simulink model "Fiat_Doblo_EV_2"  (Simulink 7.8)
settings: Solver=ode23t  StartTime=0.0  StopTime=1180  MaxStep=0.01  RelTol=1e-3
InitFcn:
  | init_FIAT_Doblo_EV
StopFcn:
  | Vyhodnoceni
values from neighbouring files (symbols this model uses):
  om_diff_ic = 0    [init_FIAT_Doblo_EV.m]
  omric = 0    [init_FIAT_Doblo_EV.m]
  t_sample = 0.1    [init_FIAT_Doblo_EV.m]
  vf0 = 0    [init_FIAT_Doblo_EV.m]
undefined symbols (not defined in the file or in its folder): Battery, Battery_Pack, BatteryData, Differential, Driveshaft, Environment, Gearbox, Motor, Powertrain, Vehicle
libraries: simulink x7, simulink_need_slupdate x1, simulink_extras x1

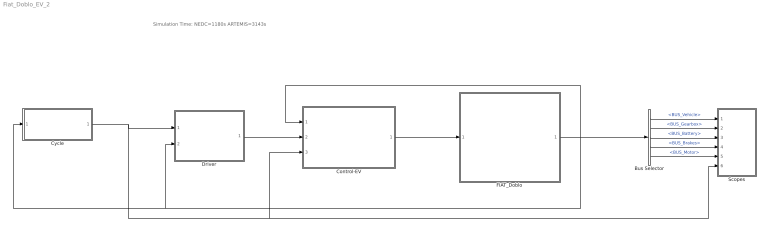
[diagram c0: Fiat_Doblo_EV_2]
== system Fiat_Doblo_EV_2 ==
  note: Simulation Time: NEDC=1180s ARTEMIS=3143s
  Bus Selector : BusSelector  OutputSignals=BUS_Vehicle,BUS_Gearbox,BUS_Battery,BUS_Brakes,BUS_Motor
  Control-EV : Subsystem
  Cycle : Subsystem
  Driver : Subsystem
  FIAT_Doblo : Subsystem
  Scopes : Subsystem
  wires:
  Control-EV/1(BUS_Control) -> FIAT_Doblo/1(BUS_Control)
  FIAT_Doblo/1(BUS_FIAT_Doblo) -> Bus Selector/1, Control-EV/1(BUS_FIAT_Doblo), Driver/2(BUS_FIAT_Doblo), Cycle/1(BUS_FIAT Doblo)
  Bus Selector/1 -> Scopes/1(BUS_Vehicle)  "<BUS_Vehicle>"
  Bus Selector/2 -> Scopes/2(BUS_Gearbox)  "<BUS_Gearbox>"
  Bus Selector/3 -> Scopes/3(BUS_Battery)  "<BUS_Battery>"
  Bus Selector/4 -> Scopes/4(BUS_Brakes)  "<BUS_Brakes>"
  Bus Selector/5 -> Scopes/5(BUS_Motor)  "<BUS_Motor>"
  Cycle/1(BUS_Cycle) -> Driver/1(BUS_Cycle), Scopes/6(BUS_Cycle), Control-EV/3(BUS_Cycle)
  Driver/1(BUS_Driver) -> Control-EV/2(BUS_Driver)

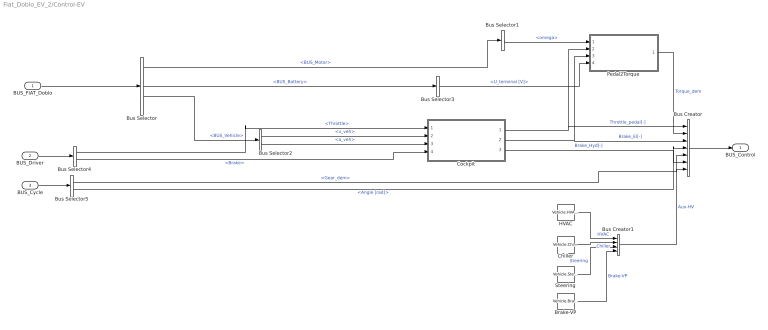
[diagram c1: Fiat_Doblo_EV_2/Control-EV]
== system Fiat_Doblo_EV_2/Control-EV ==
  BUS_FIAT_Doblo : Inport
  BUS_Driver : Inport  Port=2
  BUS_Cycle : Inport  Port=3
  Brake-VP : Constant  Value=Vehicle.BrakeVP.On
  Bus Creator : BusCreator  Inputs=7
  Bus Creator1 : BusCreator
  Bus Selector : BusSelector  OutputSignals=BUS_Motor,BUS_Gearbox,BUS_Battery,BUS_Vehicle,BUS_Brakes
  Bus Selector1 : BusSelector  OutputSignals=omega
  Bus Selector2 : BusSelector  OutputSignals=v_veh,a_veh
  Bus Selector3 : BusSelector  OutputSignals=U_terminal [V]
  Bus Selector4 : BusSelector  OutputSignals=Throttle,Brake
  Bus Selector5 : BusSelector  OutputSignals=Gear_dem,Angle [rad]
  Chiller : Constant  Value=Vehicle.Chiller.On
  Cockpit : Subsystem
  HVAC : Constant  Value=Vehicle.HVAC.On
  Pedal2Torque : Subsystem
  Steering : Constant  Value=Vehicle.Steering.On
  BUS_Control : Outport
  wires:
  Cockpit/1(Throttle1) -> Bus Creator/1, Pedal2Torque/2(Throttle_pedal[-])  "Throttle_pedal[-]"
  Cockpit/2(BrakeEl) -> Bus Creator/3, Pedal2Torque/3(Brake_el[-])  "Brake_El[-]"
  Bus Creator/1 -> BUS_Control/1
  Bus Selector2/1 -> Cockpit/2(v-veh)  "<v_veh>"
  Bus Selector2/2 -> Cockpit/3(a-veh)  "<a_veh>"
  Cockpit/3(BrakeHyd) -> Bus Creator/6  "Brake_Hyd[-]"
  HVAC/1 -> Bus Creator1/1  "HVAC"
  Chiller/1 -> Bus Creator1/2  "Chiller"
  Steering/1 -> Bus Creator1/3  "Steering"
  Brake-VP/1 -> Bus Creator1/4  "Brake-VP"
  Bus Creator1/1 -> Bus Creator/7  "Aux-HV"
  Bus Selector1/1 -> Pedal2Torque/1(om_motor)  "<omega>"
  Pedal2Torque/1(Te) -> Bus Creator/2  "Torque_dem"
  Bus Selector/3 -> Bus Selector3/1  "<BUS_Battery>"
  Bus Selector3/1 -> Pedal2Torque/4(Voltage [V])  "<U_terminal [V]>"
  BUS_FIAT_Doblo/1 -> Bus Selector/1
  Bus Selector/4 -> Bus Selector2/1  "<BUS_Vehicle>"
  Bus Selector/1 -> Bus Selector1/1  "<BUS_Motor>"
  BUS_Driver/1 -> Bus Selector4/1
  Bus Selector4/1 -> Cockpit/1(Throttle_in)  "<Throttle>"
  Bus Selector4/2 -> Cockpit/4(Brake)  "<Brake>"
  BUS_Cycle/1 -> Bus Selector5/1
  Bus Selector5/1 -> Bus Creator/5  "<Gear_dem>"
  Bus Selector5/2 -> Bus Creator/4  "<Angle [rad]>"

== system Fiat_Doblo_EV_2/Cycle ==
  BUS_FIAT Doblo : Inport
  Acc : Step  Time=15  After=250  SampleTime=0
  Bus Creator : BusCreator  Inputs=3
  Bus Selector : BusSelector  OutputSignals=BUS_Vehicle.s_veh
  Constant1 : Constant
  Constant2 : Constant  Value=2
  Constant4 : Constant  Value=0
  Demux1 : Demux  Outputs=2
  From File3 : FromFile  FileName=NEDC.mat  ExtrapolationBeforeFirstDataPoint=Hold first value  ExtrapolationAfterLastDataPoint=Hold last value  SampleTime=0.1
  From File4 : FromFile  FileName=artemis_mw130.mat  ExtrapolationBeforeFirstDataPoint=Hold first value  ExtrapolationAfterLastDataPoint=Hold last value  SampleTime=0.1
  From File5 : FromFile  FileName=artemis_URM150.mat  ExtrapolationBeforeFirstDataPoint=Hold first value  ExtrapolationAfterLastDataPoint=Hold last value  SampleTime=0.1
  Multiport Switch : MultiPortSwitch  Inputs=4  zeroidx=off
  Terminator1 : Terminator
  To Workspace : ToWorkspace  VariableName=v_dem  SampleTime=t_sample  SaveFormat=Array
  To Workspace2 : ToWorkspace  VariableName=Gear_dem  SampleTime=t_sample  SaveFormat=Array
  BUS_Cycle : Outport
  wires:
  Constant1/1 -> To Workspace2/1, Bus Creator/2  "Gear_dem"
  Bus Creator/1 -> BUS_Cycle/1
  Demux1/2 -> Terminator1/1
  Acc/1 -> Multiport Switch/5
  From File4/1 -> Multiport Switch/4
  From File5/1 -> Multiport Switch/3
  Demux1/1 -> Multiport Switch/2
  Multiport Switch/1 -> To Workspace/1, Bus Creator/1  "Speed_dem"
  Constant2/1 -> Multiport Switch/1
  From File3/1 -> Demux1/1
  BUS_FIAT Doblo/1 -> Bus Selector/1
  Constant4/1 -> Bus Creator/3  "Angle [rad]"

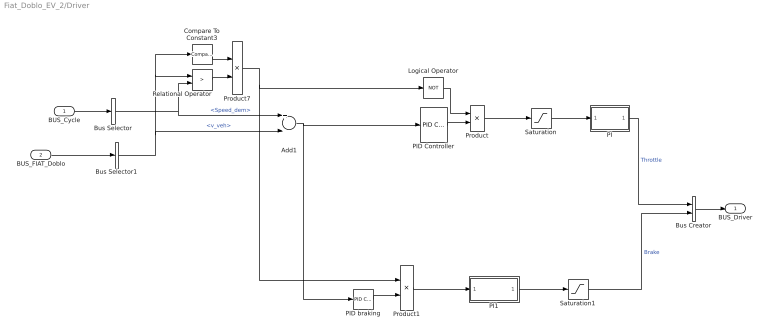
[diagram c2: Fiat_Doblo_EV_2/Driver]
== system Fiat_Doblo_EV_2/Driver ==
  BUS_Cycle : Inport
  BUS_FIAT_Doblo : Inport  Port=2
  Add1 : Sum  Inputs=+-
  Bus Creator : BusCreator  Inputs=2
  Bus Selector : BusSelector  OutputSignals=Speed_dem
  Bus Selector1 : BusSelector  OutputSignals=BUS_Vehicle.v_veh
  Compare To Constant3 : simulink/Logic and Bit Operations/Compare To Constant  relop=>  const=1  OutDataTypeStr=uint8  ZeroCross=off
  Logical Operator : Logic  Operator=NOT  AllPortsSameDT=off  OutDataTypeStr=boolean
  PI : Subsystem
  PI1 : Subsystem
  PID Controller : simulink/Continuous/PID Controller  Controller=PID  TimeDomain=Continuous-time  SampleTime=1  IntegratorMethod=Forward Euler  FilterMethod=Forward Euler  Form=Parallel  P=1  I=0.01  D=0  N=100  InitialConditionSource=internal  InitialConditionForIntegrator=0  InitialConditionForFilter=0  ExternalReset=none  LimitOutput=off  UpperSaturationLimit=1  LowerSaturationLimit=-1  LinearizeAsGain=off  AntiWindupMode=none  Kb=1  TrackingMode=off  Kt=1  PParamMin=[]  PParamMax=[]  IParamMin=[]  IParamMax=[]  DParamMin=[]  DParamMax=[]  NParamMin=[]  NParamMax=[]  KbParamMin=[]  KbParamMax=[]  KtParamMin=[]  KtParamMax=[]  POutMin=[]  POutMax=[]  IOutMin=[]  IOutMax=[]  DOutMin=[]  DOutMax=[]  NOutMin=[]  NOutMax=[]  KbOutMin=[]  KbOutMax=[]  KtOutMin=[]  KtOutMax=[]  IntegratorOutMin=[]  IntegratorOutMax=[]  FilterOutMin=[]  FilterOutMax=[]  SumOutMin=[]  SumOutMax=[]  SumI1OutMin=[]  SumI1OutMax=[]  SumI2OutMin=[]  SumI2OutMax=[]  SumI3OutMin=[]  SumI3OutMax=[]  SumDOutMin=[]  SumDOutMax=[]  SaturationOutMin=[]  SaturationOutMax=[]  IntegratorContinuousStateAttributes=''  IntegratorStateMustResolveToSignalObject=off  IntegratorRTWStateStorageClass=Auto  FilterContinuousStateAttributes=''  FilterStateMustResolveToSignalObject=off  FilterRTWStateStorageClass=Auto
  PID braking : simulink_need_slupdate/PID Controller  P=0.3  I=0.01  D=0
  Product : Product
  Product1 : Product
  Product7 : Product
  Relational Operator : RelationalOperator  Operator=>  OutDataTypeStr=boolean
  Saturation : Saturate  UpperLimit=1  LowerLimit=0
  Saturation1 : Saturate  UpperLimit=0  LowerLimit=-1
  BUS_Driver : Outport
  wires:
  PID braking/1 -> Product1/2
  Product1/1 -> PI1/1(In1)
  Add1/1 -> PID braking/1, PID Controller/1
  PID Controller/1 -> Product/2
  Product/1 -> Saturation/1
  Logical Operator/1 -> Product/1
  Saturation1/1 -> Bus Creator/2  "Brake"
  Product7/1 -> Product1/1, Logical Operator/1
  Compare To Constant3/1 -> Product7/1
  Relational Operator/1 -> Product7/2
  PI1/1(Out1) -> Saturation1/1
  Saturation/1 -> PI/1(In1)
  PI/1(Out1) -> Bus Creator/1  "Throttle"
  BUS_Cycle/1 -> Bus Selector/1
  Bus Selector/1 -> Relational Operator/2, Add1/1  "<Speed_dem>"
  BUS_FIAT_Doblo/1 -> Bus Selector1/1
  Bus Selector1/1 -> Compare To Constant3/1, Relational Operator/1, Add1/2  "<v_veh>"
  Bus Creator/1 -> BUS_Driver/1

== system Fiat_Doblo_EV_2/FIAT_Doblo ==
  BUS_Control : Inport
  01-Electric Motor : Subsystem  AncestorBlock=Powertrain/Electric Drive
  02-Gearbox : Subsystem  AncestorBlock=Powertrain/03-Gearbox
  03-Differential&Drive shaft : Subsystem  AncestorBlock=Powertrain/04-Differential&Drive shaft
  04-Vehicle : Subsystem  AncestorBlock=Powertrain/05-Vehicle
  05-Battery_Pack : Subsystem  AncestorBlock=Powertrain/Battery_Pack
  06-Hydraulic Brakes : Subsystem  AncestorBlock=Powertrain/Hydraulic Brakes  TreatAsAtomicUnit=on
  Bus Creator : BusCreator  Inputs=6
  Clock : Clock
  HV-Boardnet : Subsystem  TreatAsAtomicUnit=on
  To Workspace5 : ToWorkspace  VariableName=t  SampleTime=t_sample  SaveFormat=Array
  BUS_FIAT_Doblo : Outport
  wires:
  02-Gearbox/1(BUS_Gearbox) -> 03-Differential&Drive shaft/1(BUS_Gearbox), 01-Electric Motor/1(BUS_Gearbox), Bus Creator/2  "BUS_Gearbox"
  03-Differential&Drive shaft/1(BUS_Driveshaft) -> 02-Gearbox/2(BUS_Driveshaft), 04-Vehicle/1(BUS_Driveshaft_Front)
  04-Vehicle/1(BUS_Vehicle) -> 03-Differential&Drive shaft/2(BUS_Vehicle), Bus Creator/3  "BUS_Vehicle"
  05-Battery_Pack/1(BUS_Battery) -> 01-Electric Motor/3(BUS_Battery), Bus Creator/4  "BUS_Battery"
  06-Hydraulic Brakes/1(BUS_Brakes) -> 04-Vehicle/2(BUS_Brakes), Bus Creator/5  "BUS_Brakes"
  HV-Boardnet/1(BUS-HV-Boardnet) -> 05-Battery_Pack/2(BUS-HV-Boardnet)
  Clock/1 -> To Workspace5/1
  BUS_Control/1 -> 02-Gearbox/3(BUS_Control), 01-Electric Motor/2(BUS_Control), HV-Boardnet/1(BUS-Control), 06-Hydraulic Brakes/1(BUS_Control), 04-Vehicle/3(BUS_Control)
  01-Electric Motor/1(BUS_Motor) -> 02-Gearbox/1(BUS_Motor), 05-Battery_Pack/1(BUS_Motor), Bus Creator/1  "BUS_Motor"
  Bus Creator/1 -> BUS_FIAT_Doblo/1

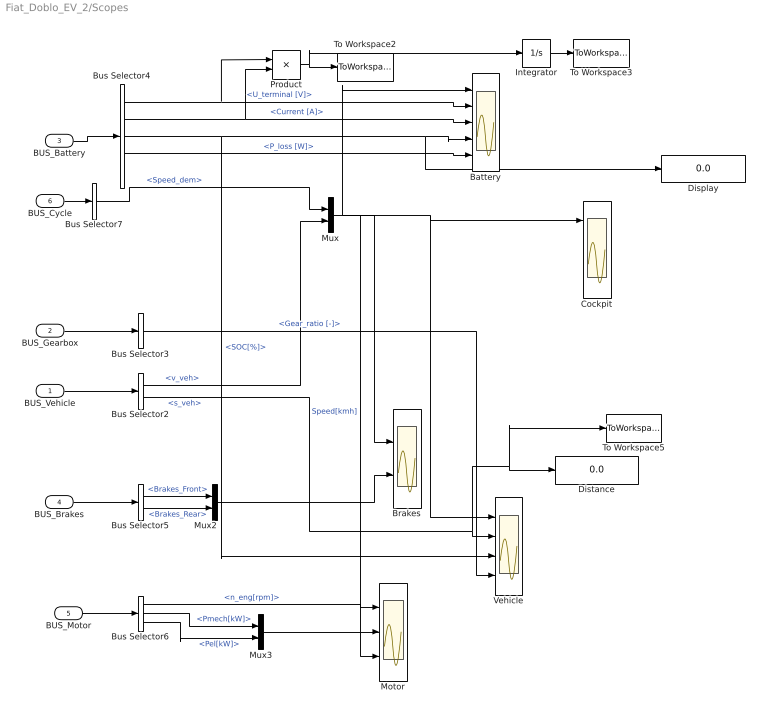
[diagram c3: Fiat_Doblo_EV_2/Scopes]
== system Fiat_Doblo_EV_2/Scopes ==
  BUS_Vehicle : Inport
  BUS_Gearbox : Inport  Port=2
  BUS_Battery : Inport  Port=3
  BUS_Brakes : Inport  Port=4
  BUS_Motor : Inport  Port=5
  BUS_Cycle : Inport  Port=6
  Battery : Scope  NumInputPorts=5
  Brakes : Scope  NumInputPorts=2
  Bus Selector2 : BusSelector  OutputSignals=v_veh,s_veh
  Bus Selector3 : BusSelector  OutputSignals=Gear_ratio [-]
  Bus Selector4 : BusSelector  OutputSignals=U_terminal [V],Current [A],SOC[%],P_loss [W],T_cell[C]
  Bus Selector5 : BusSelector  OutputSignals=Brakes_Front,Brakes_Rear
  Bus Selector6 : BusSelector  OutputSignals=n_eng[rpm],Pmech[kW],Pel[kW]
  Bus Selector7 : BusSelector  OutputSignals=Speed_dem
  Cockpit : Scope  NumInputPorts=4
  Display : Display
  Distance : Display
  Integrator : Integrator
  Motor : Scope  NumInputPorts=3
  Mux : Mux  Inputs=2
  Mux2 : Mux  Inputs=2
  Mux3 : Mux  Inputs=2
  Product : Product
  To Workspace2 : ToWorkspace  VariableName=Pbat  SampleTime=t_sample  SaveFormat=Array
  To Workspace3 : ToWorkspace  VariableName=Ebat  SampleTime=t_sample  SaveFormat=Array
  To Workspace5 : ToWorkspace  VariableName=s  SampleTime=t_sample  SaveFormat=Array
  Vehicle : Scope  NumInputPorts=4
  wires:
  BUS_Vehicle/1 -> Bus Selector2/1
  Bus Selector2/1 -> Mux/2  "<v_veh>"
  Mux/1 -> Vehicle/1, Cockpit/1, Battery/1, Brakes/1, Motor/1  "Speed[kmh]"
  Bus Selector2/2 -> Vehicle/2, Distance/1, To Workspace5/1  "<s_veh>"
  BUS_Gearbox/1 -> Bus Selector3/1
  Bus Selector3/1 -> Vehicle/4  "<Gear_ratio [-]>"
  BUS_Battery/1 -> Bus Selector4/1
  Bus Selector4/1 -> Battery/2, Product/1  "<U_terminal [V]>"
  Bus Selector4/2 -> Battery/3, Product/2  "<Current [A]>"
  Bus Selector4/3 -> Battery/4, Display/1, Vehicle/3  "<SOC[%]>"
  Bus Selector4/4 -> Battery/5  "<P_loss [W]>"
  BUS_Brakes/1 -> Bus Selector5/1
  Bus Selector5/1 -> Mux2/1  "<Brakes_Front>"
  Bus Selector5/2 -> Mux2/2  "<Brakes_Rear>"
  Mux2/1 -> Brakes/2
  BUS_Motor/1 -> Bus Selector6/1
  Bus Selector6/1 -> Motor/2  "<n_eng[rpm]>"
  Bus Selector6/2 -> Mux3/1  "<Pmech[kW]>"
  Bus Selector6/3 -> Mux3/2  "<Pel[kW]>"
  Mux3/1 -> Motor/3
  Integrator/1 -> To Workspace3/1
  Product/1 -> To Workspace2/1, Integrator/1
  BUS_Cycle/1 -> Bus Selector7/1
  Bus Selector7/1 -> Mux/1  "<Speed_dem>"

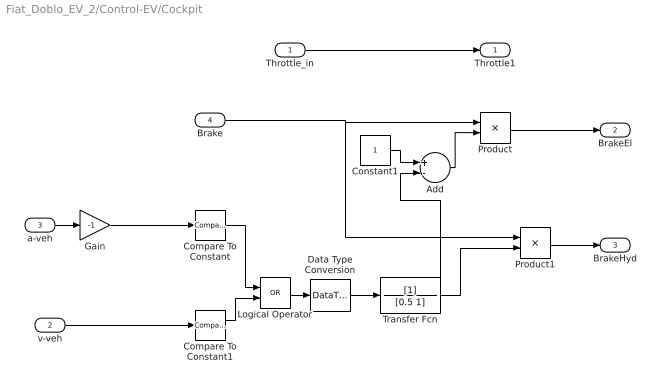
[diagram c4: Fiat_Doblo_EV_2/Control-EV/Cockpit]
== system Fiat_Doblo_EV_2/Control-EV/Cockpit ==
  Throttle_in : Inport
  v-veh : Inport  Port=2
  a-veh : Inport  Port=3
  Brake : Inport  Port=4
  Add : Sum  Inputs=+-
  Compare To Constant : simulink/Logic and Bit Operations/Compare To Constant  relop=>=  const=1  OutDataTypeStr=uint8
  Compare To Constant1 : simulink/Logic and Bit Operations/Compare To Constant  relop=<=  const=3  OutDataTypeStr=uint8
  Constant1 : Constant
  Data Type Conversion : DataTypeConversion
  Gain : Gain  Gain=-1
  Logical Operator : Logic  Operator=OR  AllPortsSameDT=off  OutDataTypeStr=boolean
  Product : Product
  Product1 : Product
  Transfer Fcn : TransferFcn  Denominator=[0.5 1]
  Throttle1 : Outport
  BrakeEl : Outport  Port=2
  BrakeHyd : Outport  Port=3
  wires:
  Throttle_in/1 -> Throttle1/1
  Product/1 -> BrakeEl/1
  Brake/1 -> Product/1, Product1/1
  Product1/1 -> BrakeHyd/1
  a-veh/1 -> Gain/1
  Add/1 -> Product/2
  Constant1/1 -> Add/1
  Gain/1 -> Compare To Constant/1
  Compare To Constant/1 -> Logical Operator/1
  v-veh/1 -> Compare To Constant1/1
  Compare To Constant1/1 -> Logical Operator/2
  Logical Operator/1 -> Data Type Conversion/1
  Transfer Fcn/1 -> Product1/2, Add/2
  Data Type Conversion/1 -> Transfer Fcn/1

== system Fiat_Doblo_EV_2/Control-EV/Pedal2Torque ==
  om_motor : Inport
  Throttle_pedal[-] : Inport  Port=2
  Brake_el[-] : Inport  Port=3
  Voltage [V] : Inport  Port=4
  1-D Lookup Table : Lookup_n-D  BreakpointsForDimension1=Motor.Maps.vector_speed  BreakpointsForDimension2=Motor.Maps.vector_voltage  Table=Motor.Maps.vector_max_torque  ExtrapMethod=Clip  UseLastTableValue=on  RndMeth=Simplest
  1-D Lookup Table1 : Lookup_n-D  BreakpointsForDimension1=Motor.Maps.vector_speed  BreakpointsForDimension2=Motor.Maps.vector_voltage  Table=Motor.Maps.vector_min_torque  ExtrapMethod=Clip  UseLastTableValue=on  RndMeth=Simplest
  Add : Sum
  Gain : Gain  Gain=-1
  Gain1 : Gain
  Product1 : Product
  Product2 : Product
  Te : Outport
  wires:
  Gain1/1 -> Add/1
  Gain/1 -> Add/2
  Product1/1 -> Gain/1
  Product2/1 -> Gain1/1
  1-D Lookup Table1/1 -> Product1/2
  1-D Lookup Table/1 -> Product2/1
  om_motor/1 -> 1-D Lookup Table1/1, 1-D Lookup Table/1
  Throttle_pedal[-]/1 -> Product2/2
  Add/1 -> Te/1
  Brake_el[-]/1 -> Product1/1
  Voltage [V]/1 -> 1-D Lookup Table1/2, 1-D Lookup Table/2

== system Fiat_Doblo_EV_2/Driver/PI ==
  In1 : Inport
  Add3 : Sum  Inputs=+-
  Constant : Constant  Value=2
  Integrator1 : Integrator
  Product1 : Product
  Out1 : Outport
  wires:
  Add3/1 -> Product1/1
  Product1/1 -> Integrator1/1
  In1/1 -> Add3/1
  Integrator1/1 -> Add3/2, Out1/1
  Constant/1 -> Product1/2

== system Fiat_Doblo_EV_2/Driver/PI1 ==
  In1 : Inport
  Add3 : Sum  Inputs=+-
  Constant : Constant
  Integrator1 : Integrator
  Product1 : Product
  Out1 : Outport
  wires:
  Constant/1 -> Product1/2
  Integrator1/1 -> Out1/1, Add3/2
  In1/1 -> Add3/1
  Product1/1 -> Integrator1/1
  Add3/1 -> Product1/1

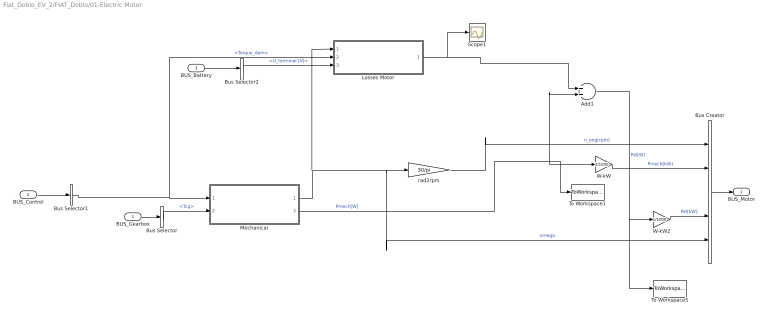
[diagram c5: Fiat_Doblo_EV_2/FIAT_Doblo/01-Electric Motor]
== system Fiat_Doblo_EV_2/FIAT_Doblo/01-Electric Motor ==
  BUS_Gearbox : Inport
  BUS_Control : Inport  Port=2
  BUS_Battery : Inport  Port=3
  Add1 : Sum
  Bus Creator : BusCreator  Inputs=5
  Bus Selector : BusSelector  OutputSignals=Tcg,om_inp
  Bus Selector1 : BusSelector  OutputSignals=Torque_dem
  Bus Selector2 : BusSelector  OutputSignals=U_terminal [V]
  Losses Motor : Subsystem
  Mechanical : Subsystem
  Scope1 : Scope
  To Workspace1 : ToWorkspace  VariableName=P_Mot_mech  SampleTime=t_sample  SaveFormat=Array
  To Workspace5 : ToWorkspace  VariableName=P_Mot_el  SampleTime=t_sample  SaveFormat=Array
  W-kW : Gain  Gain=1/1000
  W-kW2 : Gain  Gain=1/1000
  rad2rpm : Gain  Gain=30/pi
  BUS_Motor : Outport
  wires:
  W-kW2/1 -> Bus Creator/4  "Pel[kW]"
  W-kW/1 -> Bus Creator/2  "Pmech[kW]"
  Add1/1 -> W-kW2/1, To Workspace5/1  "Pel[W]"
  Losses Motor/1(P_loss) -> Scope1/1, Add1/1
  BUS_Control/1 -> Bus Selector1/1
  Bus Selector/1 -> Mechanical/2(Tcg)  "<Tcg>"
  BUS_Gearbox/1 -> Bus Selector/1
  Bus Creator/1 -> BUS_Motor/1
  Mechanical/2(Pmech) -> W-kW/1, Add1/2, To Workspace1/1  "Pmech[W]"
  Mechanical/1(om_e) -> rad2rpm/1, Bus Creator/5, Losses Motor/1(Speed)  "omega"
  rad2rpm/1 -> Bus Creator/1  "n_eng[rpm]"
  BUS_Battery/1 -> Bus Selector2/1
  Bus Selector2/1 -> Losses Motor/3(Voltage [V])  "<U_terminal [V]>"
  Bus Selector1/1 -> Mechanical/1(Te), Losses Motor/2(Torque)  "<Torque_dem>"

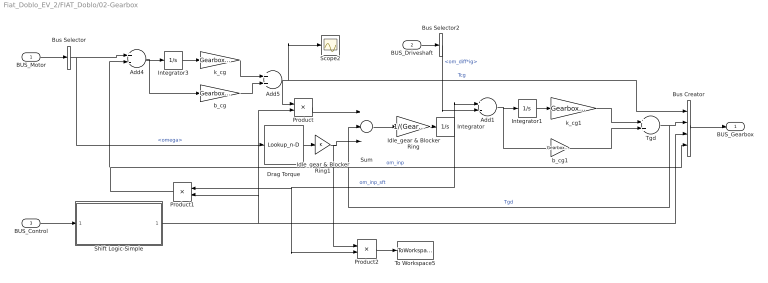
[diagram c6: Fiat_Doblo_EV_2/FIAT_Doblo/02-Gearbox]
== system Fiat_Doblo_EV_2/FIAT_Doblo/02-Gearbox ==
  BUS_Motor : Inport
  BUS_Driveshaft : Inport  Port=2
  BUS_Control : Inport  Port=3
  Add1 : Sum  Inputs=+-
  Add4 : Sum  Inputs=+-
  Add5 : Sum
  Bus Creator : BusCreator
  Bus Selector : BusSelector  OutputSignals=omega
  Bus Selector2 : BusSelector  OutputSignals=om_diff*ig
  Drag Torque : Lookup_n-D  NumberOfTableDimensions=1  BreakpointsForDimension1=Gearbox.Vector.Speed  Table=Gearbox.Vector.DragTorque  RndMeth=Simplest
  Idle_gear & Blocker Ring : Gain  Gain=1/(Gearbox.Inpsft.Inertia+Gearbox.Outpsft.Inertia)
  Idle_gear & Blocker Ring1 : Gain
  Integrator : Integrator
  Integrator1 : Integrator
  Integrator3 : Integrator
  Product : Product
  Product1 : Product
  Product2 : Product
  Scope2 : Scope
  Shift Logic-Simple : Subsystem
  Sum : Sum  Inputs=+--
  Tgd : Sum
  To Workspace5 : ToWorkspace  VariableName=P_Gearbox  SampleTime=t_sample  SaveFormat=Array
  b_cg : Gain  Gain=Gearbox.Inpsft.b
  b_cg1 : Gain  Gain=Gearbox.Outpsft.b
  k_cg : Gain  Gain=Gearbox.Inpsft.c
  k_cg1 : Gain  Gain=Gearbox.Outpsft.c
  BUS_Gearbox : Outport
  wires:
  Drag Torque/1 -> Idle_gear & Blocker Ring1/1
  Bus Selector2/1 -> Add1/2  "<om_diff*ig>"
  BUS_Driveshaft/1 -> Bus Selector2/1
  Tgd/1 -> Bus Creator/2, Sum/2  "Tgd"
  Add1/1 -> b_cg1/1, Integrator1/1
  Integrator1/1 -> k_cg1/1
  k_cg1/1 -> Tgd/1
  b_cg1/1 -> Tgd/2
  Shift Logic-Simple/1(Gear_ratio) -> Bus Creator/3, Product1/2, Product/2
  Bus Creator/1 -> BUS_Gearbox/1
  BUS_Control/1 -> Shift Logic-Simple/1(BUS_Control)
  Bus Selector/1 -> Add4/1, Drag Torque/1  "<omega>"
  BUS_Motor/1 -> Bus Selector/1
  Product1/1 -> Add4/2, Bus Creator/4  "om_inp"
  Product/1 -> Sum/1
  b_cg/1 -> Add5/2
  k_cg/1 -> Add5/1
  Integrator3/1 -> k_cg/1
  Add4/1 -> Integrator3/1, b_cg/1
  Integrator/1 -> Add1/1, Product1/1, Product2/2  "om_inp_sft"
  Idle_gear & Blocker Ring/1 -> Integrator/1
  Sum/1 -> Idle_gear & Blocker Ring/1
  Add5/1 -> Product/1, Bus Creator/1, Scope2/1  "Tcg"
  Product2/1 -> To Workspace5/1
  Idle_gear & Blocker Ring1/1 -> Sum/3, Product2/1

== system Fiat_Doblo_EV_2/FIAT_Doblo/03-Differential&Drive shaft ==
  BUS_Gearbox : Inport
  BUS_Vehicle : Inport  Port=2
  Bus Creator : BusCreator  Inputs=2
  Bus Selector2 : BusSelector  OutputSignals=Tgd
  Differential : Subsystem
  Driveshafts : Subsystem
  BUS_Driveshaft : Outport
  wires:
  Driveshafts/1(T_drvsft) -> Differential/2(T_drv_sft), Bus Creator/1
  Differential/2(om_diff*ig) -> Bus Creator/2  "om_diff*ig"
  Bus Selector2/1 -> Differential/1(Tgd)  "<Tgd>"
  Differential/1(om_diff) -> Driveshafts/1(om_diff)
  BUS_Vehicle/1 -> Driveshafts/2(BUS_Vehicle)
  Bus Creator/1 -> BUS_Driveshaft/1
  BUS_Gearbox/1 -> Bus Selector2/1

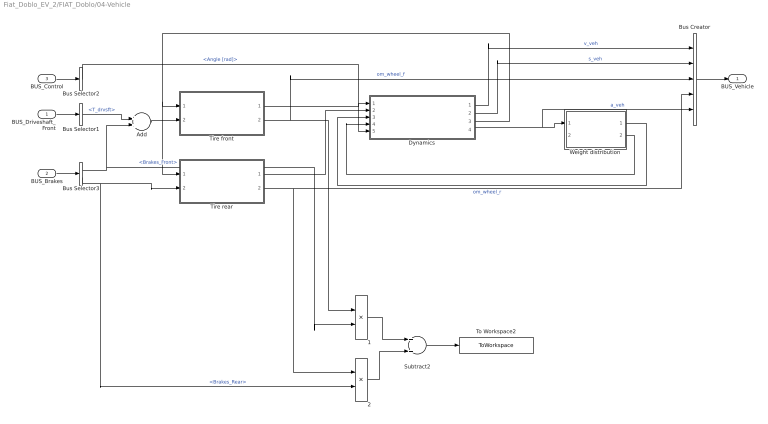
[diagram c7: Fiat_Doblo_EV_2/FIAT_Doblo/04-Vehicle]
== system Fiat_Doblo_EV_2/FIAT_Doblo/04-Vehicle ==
  BUS_Driveshaft_Front : Inport
  BUS_Brakes : Inport  Port=2
  BUS_Control : Inport  Port=3
  "          1" : Product  Inputs=**
  "          2" : Product  Inputs=**
  Add : Sum
  Bus Creator : BusCreator  Inputs=5
  Bus Selector1 : BusSelector  OutputSignals=T_drvsft
  Bus Selector2 : BusSelector  OutputSignals=Angle [rad]
  Bus Selector3 : BusSelector  OutputSignals=Brakes_Front,Brakes_Rear
  Dynamics : Subsystem
  Subtract2 : Sum
  Tire front : Subsystem
  Tire rear : Subsystem
  To Workspace2 : ToWorkspace  VariableName=P_brakes  SampleTime=t_sample  SaveFormat=Array
  Weight distribution : Subsystem
  BUS_Vehicle : Outport
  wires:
  Tire rear/2(om_wheel) -> Bus Creator/4, "          2"/1  "om_wheel_r"
  Tire front/2(om_wheel) -> Bus Creator/3, "          1"/1  "om_wheel_f"
  Dynamics/4(Acc) -> Weight distribution/1(acc), Bus Creator/5  "a_veh"
  Dynamics/3(v_f[m/s]) -> Tire rear/1(v_f), Tire front/1(v_f)
  Dynamics/1(v_veh) -> Bus Creator/1  "v_veh"
  Weight distribution/2(Fn_Wheel_R) -> Dynamics/4(Fn_Wheel_R)
  Weight distribution/1(Fn_Wheel_F) -> Dynamics/3(Fn_Wheel_F)
  Bus Creator/1 -> BUS_Vehicle/1
  BUS_Driveshaft_Front/1 -> Bus Selector1/1
  Tire rear/1(F_tire) -> Dynamics/2(F_tire_rear)
  Tire front/1(F_tire) -> Dynamics/1(F_tire_front)
  Dynamics/2(s_veh) -> Bus Creator/2  "s_veh"
  Add/1 -> Tire front/2(T_drsft)
  Bus Selector1/1 -> Add/1  "<T_drvsft>"
  BUS_Brakes/1 -> Bus Selector3/1
  Bus Selector3/1 -> Add/2, "          1"/2  "<Brakes_Front>"
  Bus Selector3/2 -> "          2"/2, Tire rear/2(T_drsft)  "<Brakes_Rear>"
  "          1"/1 -> Subtract2/1
  Subtract2/1 -> To Workspace2/1
  "          2"/1 -> Subtract2/2
  BUS_Control/1 -> Bus Selector2/1
  Bus Selector2/1 -> Dynamics/5(Road_Incline[rad])  "<Angle [rad]>"

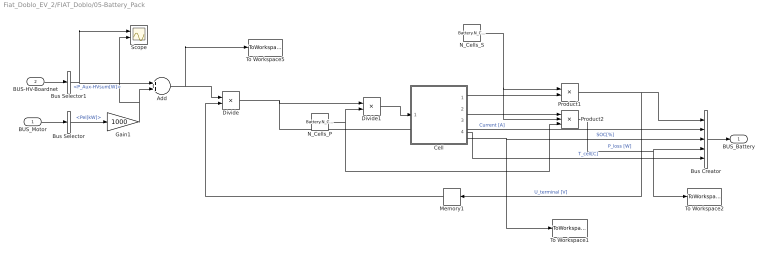
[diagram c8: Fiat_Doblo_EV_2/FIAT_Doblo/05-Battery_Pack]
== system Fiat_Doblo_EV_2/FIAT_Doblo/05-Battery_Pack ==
  BUS_Motor : Inport
  BUS-HV-Boardnet : Inport  Port=2
  Add : Sum
  Bus Creator : BusCreator  Inputs=5
  Bus Selector : BusSelector  OutputSignals=Pel[kW]
  Bus Selector1 : BusSelector  OutputSignals=P_Aux-HVsum[W]
  Cell : Subsystem
  Divide : Product  Inputs=*/
  Divide1 : Product  Inputs=*/
  Gain1 : Gain  Gain=1000
  Memory1 : Memory  X0=400
  N_Cells_P : Constant  Value=Battery.N_Cells.P
  N_Cells_S : Constant  Value=Battery.N_Cells.S
  Product1 : Product
  Product2 : Product  Inputs=3
  Scope : Scope  NumInputPorts=2
  To Workspace1 : ToWorkspace  VariableName=SOC  SampleTime=t_sample  SaveFormat=Array
  To Workspace2 : ToWorkspace  VariableName=P_Batt_loss  SampleTime=t_sample  SaveFormat=Array
  To Workspace5 : ToWorkspace  VariableName=P_Batt  SampleTime=t_sample  SaveFormat=Array
  BUS_Battery : Outport
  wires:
  Memory1/1 -> Divide/2
  Cell/4(T_cell[C]) -> Bus Creator/5  "T_cell[C]"
  Product2/1 -> Bus Creator/4, To Workspace2/1  "P_loss [W]"
  Cell/3(SOC[%]) -> Bus Creator/3, To Workspace1/1  "SOC[%]"
  Divide1/1 -> Cell/1(Current [A])
  N_Cells_P/1 -> Product2/3, Divide1/2
  Divide/1 -> Divide1/1, Bus Creator/2  "Current [A]"
  Cell/2(P_loss [w]) -> Product2/1
  N_Cells_S/1 -> Product2/2, Product1/1
  Cell/1(U_terminal [V]) -> Product1/2
  Product1/1 -> Memory1/1, Bus Creator/1  "U_terminal [V]"
  Bus Selector/1 -> Gain1/1  "<Pel[kW]>"
  BUS_Motor/1 -> Bus Selector/1
  Bus Creator/1 -> BUS_Battery/1
  BUS-HV-Boardnet/1 -> Bus Selector1/1
  Bus Selector1/1 -> Add/1, Scope/1  "<P_Aux-HVsum[W]>"
  Gain1/1 -> Add/2, Scope/2
  Add/1 -> Divide/1, To Workspace5/1

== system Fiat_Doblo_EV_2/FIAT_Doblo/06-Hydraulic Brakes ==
  BUS_Control : Inport
  Bus Creator : BusCreator  Inputs=2
  Bus Selector : BusSelector  OutputSignals=Brake_Hyd[-]
  Gain1 : Gain  Gain=0.6
  Gain2 : Gain  Gain=0.4
  Pos2Nm : Gain  Gain=800
  BUS_Brakes : Outport
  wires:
  Bus Selector/1 -> Pos2Nm/1  "<Brake_Hyd[-]>"
  BUS_Control/1 -> Bus Selector/1
  Gain1/1 -> Bus Creator/1  "Brakes_Front"
  Gain2/1 -> Bus Creator/2  "Brakes_Rear"
  Bus Creator/1 -> BUS_Brakes/1
  Pos2Nm/1 -> Gain1/1, Gain2/1

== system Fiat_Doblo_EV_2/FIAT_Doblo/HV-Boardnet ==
  BUS-Control : Inport
  Add : Sum  Inputs=++++
  Brake-VP : Constant  Value=Vehicle.BrakeVP.Power
  Bus Creator : BusCreator  Inputs=5
  Bus Selector : BusSelector  OutputSignals=Aux-HV.HVAC,Aux-HV.Chiller,Aux-HV.Steering,Aux-HV.Brake-VP
  Chiller : Constant  Value=Vehicle.Chiller.Power
  HVAC : Constant  Value=Vehicle.HVAC.Power
  Product{,1..3} (4 alike) : Product
  Steering : Constant  Value=Vehicle.Steering.Power
  To Workspace2 : ToWorkspace  VariableName=P_Aux  SampleTime=t_sample  SaveFormat=Array
  BUS-HV-Boardnet : Outport
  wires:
  HVAC/1 -> Product/2
  Chiller/1 -> Product1/2
  Steering/1 -> Product2/2
  Brake-VP/1 -> Product3/2
  BUS-Control/1 -> Bus Selector/1
  Bus Creator/1 -> BUS-HV-Boardnet/1
  Product/1 -> Bus Creator/1, Add/1  "P_HVAC[W]"
  Product1/1 -> Bus Creator/2, Add/2  "P_Chiller[W]"
  Product2/1 -> Bus Creator/3, Add/3  "P_Steering[W]"
  Product3/1 -> Bus Creator/4, Add/4  "P_Brake-VP[W]"
  Bus Selector/1 -> Product/1  "<HVAC>"
  Bus Selector/2 -> Product1/1  "<Chiller>"
  Bus Selector/3 -> Product2/1  "<Steering>"
  Bus Selector/4 -> Product3/1  "<Brake-VP>"
  Add/1 -> Bus Creator/5, To Workspace2/1  "P_Aux-HVsum[W]"

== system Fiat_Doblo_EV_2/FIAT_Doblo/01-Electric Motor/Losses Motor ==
  Speed : Inport
  Torque : Inport  Port=2
  Voltage [V] : Inport  Port=3
  2-D Lookup Table : Lookup_n-D  NumberOfTableDimensions=3  BreakpointsForDimension1=Motor.Maps.vector_speed  BreakpointsForDimension2=Motor.Maps.vector_torque  BreakpointsForDimension3=Motor.Maps.vector_voltage  Table=Motor.Maps.map_ploss  ExtrapMethod=Clip  RemoveProtectionInput=on  UseLastTableValue=on  RndMeth=Simplest
  Abs : Abs
  P_loss : Outport
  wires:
  Abs/1 -> P_loss/1
  2-D Lookup Table/1 -> Abs/1
  Speed/1 -> 2-D Lookup Table/1
  Torque/1 -> 2-D Lookup Table/2
  Voltage [V]/1 -> 2-D Lookup Table/3

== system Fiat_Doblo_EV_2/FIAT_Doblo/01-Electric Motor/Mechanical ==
  Te : Inport
  Tcg : Inport  Port=2
  Add1 : Sum  Inputs=+-
  Gain : Gain  Gain=1/Motor.Inertia
  Integrator : Integrator
  Product : Product
  om_e : Outport
  Pmech : Outport  Port=2
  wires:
  Te/1 -> Product/2, Add1/1
  Product/1 -> Pmech/1
  Integrator/1 -> Product/1, om_e/1  "om_e"
  Gain/1 -> Integrator/1
  Add1/1 -> Gain/1
  Tcg/1 -> Add1/2

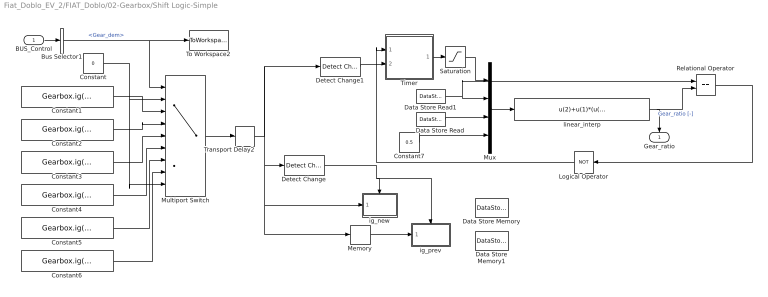
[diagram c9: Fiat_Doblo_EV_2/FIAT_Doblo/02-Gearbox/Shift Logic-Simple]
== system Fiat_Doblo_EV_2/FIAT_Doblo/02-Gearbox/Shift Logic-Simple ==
  BUS_Control : Inport
  Bus Selector1 : BusSelector  OutputSignals=Gear_dem
  Constant : Constant  Value=0
  Constant1 : Constant  Value=Gearbox.ig(1)
  Constant2 : Constant  Value=Gearbox.ig(2)
  Constant3 : Constant  Value=Gearbox.ig(3)
  Constant4 : Constant  Value=Gearbox.ig(4)
  Constant5 : Constant  Value=Gearbox.ig(5)
  Constant6 : Constant  Value=Gearbox.ig(6)
  Constant7 : Constant  Value=0.5
  Data Store Memory : DataStoreMemory  DataStoreName=ig_new
  Data Store Memory1 : DataStoreMemory  DataStoreName=ig_prev
  Data Store Read : DataStoreRead  DataStoreName=ig_new  SampleTime=0
  Data Store Read1 : DataStoreRead  DataStoreName=ig_prev  SampleTime=0
  Detect Change : simulink/Logic and Bit Operations/Detect Change  vinit=0  InputProcessing=Inherited  OutDataTypeStr=uint8
  Detect Change1 : simulink/Logic and Bit Operations/Detect Change  vinit=0  InputProcessing=Inherited  OutDataTypeStr=boolean
  Logical Operator : Logic  Operator=NOT  AllPortsSameDT=off  OutDataTypeStr=boolean
  Memory : Memory
  Multiport Switch : MultiPortSwitch  DataPortOrder=Zero-based contiguous  Inputs=7  DataPortForDefault=Additional data port  zeroidx=on
  Mux : Mux
  Relational Operator : RelationalOperator  Operator===  OutDataTypeStr=boolean
  Saturation : Saturate  LowerLimit=0
  Timer : Subsystem
  To Workspace2 : ToWorkspace  VariableName=Gear  SampleTime=t_sample  SaveFormat=Array
  Transport Delay2 : TransportDelay  DelayTime=0.3  BufferSize=10000
  ig_new : Subsystem  TreatAsAtomicUnit=on
  ig_prev : Subsystem  TreatAsAtomicUnit=on
  linear_interp : Fcn  Expr=u(2)+u(1)*(u(3)-u(2))/u(4)
  Gear_ratio : Outport
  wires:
  BUS_Control/1 -> Bus Selector1/1
  Transport Delay2/1 -> Detect Change1/1, Memory/1, ig_new/1(ig), Detect Change/1
  Saturation/1 -> Mux/1
  Logical Operator/1 -> Timer/1(Set)
  Detect Change1/1 -> Timer/2(Reset)
  Relational Operator/1 -> Logical Operator/1
  linear_interp/1 -> Gear_ratio/1, Relational Operator/2  "Gear_ratio [-]"
  Constant7/1 -> Mux/4
  Data Store Read/1 -> Mux/3
  Data Store Read1/1 -> Mux/2, Relational Operator/1
  Timer/1(Count) -> Saturation/1
  Memory/1 -> ig_prev/1(ig)
  Detect Change/1 -> ig_prev/Trigger, ig_new/Trigger
  Mux/1 -> linear_interp/1
  Constant/1 -> Multiport Switch/9, Multiport Switch/2
  Constant6/1 -> Multiport Switch/8
  Constant5/1 -> Multiport Switch/7
  Constant4/1 -> Multiport Switch/6
  Constant3/1 -> Multiport Switch/5
  Constant2/1 -> Multiport Switch/4
  Constant1/1 -> Multiport Switch/3
  Bus Selector1/1 -> Multiport Switch/1, To Workspace2/1  "<Gear_dem>"
  Multiport Switch/1 -> Transport Delay2/1

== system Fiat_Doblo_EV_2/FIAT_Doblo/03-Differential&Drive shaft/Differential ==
  Tgd : Inport
  T_drv_sft : Inport  Port=2
  Gain : Gain  Gain=Differential.ig(1)
  Sum5 : Sum  Inputs=+-|
  inertia rear drive shaft : Gain  Gain=1/Differential.Inertia
  ratio target gear : Gain  Gain=Differential.ig(1)
  "to_angle " : Integrator  InitialCondition=om_diff_ic
  om_diff : Outport
  om_diff*ig : Outport  Port=2
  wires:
  Gain/1 -> om_diff*ig/1
  Tgd/1 -> ratio target gear/1
  ratio target gear/1 -> Sum5/1  "T_outp_sft_i"
  "to_angle "/1 -> Gain/1, om_diff/1  "om_diff [rad/s]"
  Sum5/1 -> inertia rear drive shaft/1
  inertia rear drive shaft/1 -> "to_angle "/1  "omp_diff"
  T_drv_sft/1 -> Sum5/2  "T_drv_sft"

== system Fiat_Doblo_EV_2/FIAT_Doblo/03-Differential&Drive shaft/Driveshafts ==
  om_diff : Inport
  BUS_Vehicle : Inport  Port=2
  Add4 : Sum  Inputs=+-
  Add5 : Sum
  Bus Selector1 : BusSelector  OutputSignals=om_wheel_f
  Integrator3 : Integrator
  To Workspace1 : ToWorkspace  VariableName=T_drvsft  SampleTime=t_sample  SaveFormat=Array
  b_cg : Gain  Gain=Driveshaft.Left.b+Driveshaft.Right.b
  k_cg : Gain  Gain=Driveshaft.Left.c+Driveshaft.Right.c
  T_drvsft : Outport
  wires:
  BUS_Vehicle/1 -> Bus Selector1/1
  om_diff/1 -> Add4/1
  Add5/1 -> T_drvsft/1, To Workspace1/1  "T_drvsft"
  b_cg/1 -> Add5/2
  k_cg/1 -> Add5/1
  Integrator3/1 -> k_cg/1
  Add4/1 -> Integrator3/1, b_cg/1
  Bus Selector1/1 -> Add4/2  "<om_wheel_f>"

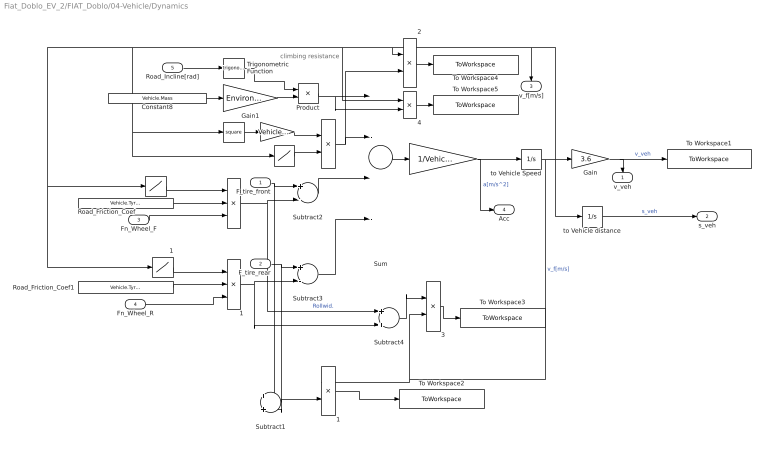
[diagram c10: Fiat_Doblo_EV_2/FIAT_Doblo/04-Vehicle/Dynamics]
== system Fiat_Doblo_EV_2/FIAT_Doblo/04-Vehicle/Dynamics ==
  note: climbing resistance
  F_tire_front : Inport
  F_tire_rear : Inport  Port=2
  Fn_Wheel_F : Inport  Port=3
  Fn_Wheel_R : Inport  Port=4
  Road_Incline[rad] : Inport  Port=5
  "  " : Gain  Gain=1/Vehicle.Mass
  "     " : Gain  Gain=Vehicle.cx*Vehicle.AreaF*Environment.Air.ro*0.5
  "      " : Math  Operator=square
  "        " : Product  Inputs=***
  "         " : Lookup  InputValues=[-1 -0.01 0 0.01 1]  Table=[-1 -1 0 1 1]
            {,1..4} (5 alike) : Product  Inputs=**
  "            " : Lookup  InputValues=[-1 -0.01 0 0.01 1]  Table=[-1 -1 0 1 1]
  "         1" : Lookup  InputValues=[-1 -0.01 0 0.01 1]  Table=[-1 -1 0 1 1]
  "        1" : Product  Inputs=***
  Constant8 : Constant  Value=Vehicle.Mass
  Gain : Gain  Gain=3.6
  Gain1 : Gain  Gain=Environment.g
  Product : Product
  Road_Friction_Coef : Constant  Value=Vehicle.Tyre.Front.f
  Road_Friction_Coef1 : Constant  Value=Vehicle.Tyre.Rear.f
  Subtract1 : Sum
  Subtract2 : Sum  Inputs=+-
  Subtract3 : Sum  Inputs=+-
  Subtract4 : Sum
  Sum : Sum  Inputs=|-|-|+|+
  To Workspace1 : ToWorkspace  VariableName=v_vehicle  SampleTime=t_sample  SaveFormat=Array
  To Workspace2 : ToWorkspace  VariableName=P_vehicle  SampleTime=t_sample  SaveFormat=Array
  To Workspace3 : ToWorkspace  VariableName=P_roll  SampleTime=t_sample  SaveFormat=Array
  To Workspace4 : ToWorkspace  VariableName=P_air  SampleTime=t_sample  SaveFormat=Array
  To Workspace5 : ToWorkspace  VariableName=P_climb  SampleTime=t_sample  SaveFormat=Array
  Trigonometric Function : Trigonometry
  to Vehicle Speed : Integrator  InitialCondition=vf0
  to Vehicle distance : Integrator  InitialCondition=vf0
  v_veh : Outport
  s_veh : Outport  Port=2
  v_f[m/s] : Outport  Port=3
  Acc : Outport  Port=4
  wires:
  Fn_Wheel_R/1 -> "        1"/3
  F_tire_rear/1 -> Subtract3/1, Subtract1/2
  Fn_Wheel_F/1 -> "        "/3
  F_tire_front/1 -> Subtract2/1, Subtract1/1
  to Vehicle distance/1 -> s_veh/1  "s_veh"
  Product/1 -> Sum/1, "          4"/2
  Constant8/1 -> Gain1/1
  "        1"/1 -> Subtract3/2, Subtract4/2
  Subtract3/1 -> Sum/4
  Road_Friction_Coef1/1 -> "        1"/2
  "         1"/1 -> "        1"/1
  "        "/1 -> Subtract2/2, Subtract4/1  "Rollwid."
  Subtract2/1 -> Sum/3
  Gain/1 -> v_veh/1, To Workspace1/1  "v_veh"
  to Vehicle Speed/1 -> v_f[m/s]/1, "          2"/1, "         1"/1, "         "/1, "            "/1, "      "/1, "          4"/1, to Vehicle distance/1, Gain/1, "          1"/1, "          3"/2  "v_f[m/s]"
  "  "/1 -> Acc/1, to Vehicle Speed/1  "a[m/s^2]"
  "            "/1 -> "          "/2
  "     "/1 -> "          "/1
  "          "/1 -> Sum/2, "          2"/2
  Road_Friction_Coef/1 -> "        "/2
  "         "/1 -> "        "/1
  "      "/1 -> "     "/1
  Sum/1 -> "  "/1
  "          1"/1 -> To Workspace2/1
  Subtract1/1 -> "          1"/2
  "          2"/1 -> To Workspace4/1
  Subtract4/1 -> "          3"/1
  "          3"/1 -> To Workspace3/1
  Gain1/1 -> Product/2
  Road_Incline[rad]/1 -> Trigonometric Function/1
  Trigonometric Function/1 -> Product/1
  "          4"/1 -> To Workspace5/1

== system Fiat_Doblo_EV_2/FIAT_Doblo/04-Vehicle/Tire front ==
  v_f : Inport
  T_drsft : Inport  Port=2
  "            " : Gain  Gain=2
  "            1" : Gain  Gain=Vehicle.Tyre.Front.c
  "            2" : Gain  Gain=Vehicle.Tyre.Front.Rdyn
  "            3" : Gain  Gain=Vehicle.Tyre.Front.b
  Sum1 : Sum  Inputs=2
  Sum10 : Sum  Inputs=+-
  To Workspace1 : ToWorkspace  VariableName=om_wheel  SampleTime=t_sample  SaveFormat=Array
  Wheel : Subsystem
  "to Rot Speed     " : Integrator
  F_tire : Outport
  om_wheel : Outport  Port=2
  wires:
  "            3"/1 -> Sum1/2
  "            1"/1 -> Sum1/1  "[N]"
  Sum10/1 -> "            3"/1, "to Rot Speed     "/1
  "            2"/1 -> Sum10/1
  "to Rot Speed     "/1 -> "            1"/1
  v_f/1 -> Sum10/2
  Wheel/1(om_wheel) -> To Workspace1/1, om_wheel/1, "            2"/1  "om_wheel [1/s]"
  Sum1/1 -> Wheel/1(F_tire), "            "/1  "[N]"
  "            "/1 -> F_tire/1  "F_tire [N]"
  T_drsft/1 -> Wheel/2(T_drsft)  "T_drv_sft"

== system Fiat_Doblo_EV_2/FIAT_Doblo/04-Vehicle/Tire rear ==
  v_f : Inport
  T_drsft : Inport  Port=2
  "            " : Gain  Gain=2
  "            1" : Gain  Gain=Vehicle.Tyre.Front.c
  "            2" : Gain  Gain=Vehicle.Tyre.Front.Rdyn
  "            3" : Gain  Gain=Vehicle.Tyre.Front.b
  Sum1 : Sum  Inputs=2
  Sum10 : Sum  Inputs=+-
  To Workspace1 : ToWorkspace  VariableName=om_wheel2  SampleTime=t_sample  SaveFormat=Array
  Wheel : Subsystem
  "to Rot Speed     " : Integrator
  F_tire : Outport
  om_wheel : Outport  Port=2
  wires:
  T_drsft/1 -> Wheel/2(T_drsft)  "T_drv_sft"
  "            "/1 -> F_tire/1  "F_tire [N]"
  Sum1/1 -> "            "/1, Wheel/1(F_tire)  "[N]"
  Wheel/1(om_wheel) -> om_wheel/1, To Workspace1/1, "            2"/1  "om_wheel [1/s]"
  v_f/1 -> Sum10/2
  "to Rot Speed     "/1 -> "            1"/1
  "            2"/1 -> Sum10/1
  Sum10/1 -> "to Rot Speed     "/1, "            3"/1
  "            1"/1 -> Sum1/1  "[N]"
  "            3"/1 -> Sum1/2

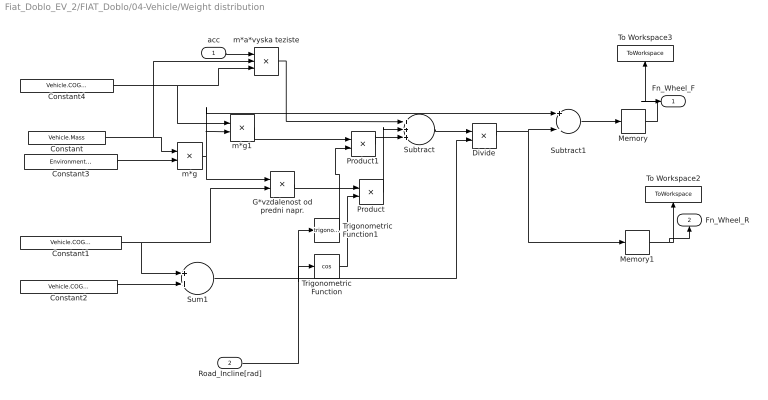
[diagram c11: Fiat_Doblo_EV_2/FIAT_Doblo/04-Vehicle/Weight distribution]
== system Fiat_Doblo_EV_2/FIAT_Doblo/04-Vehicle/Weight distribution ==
  acc : Inport
  Road_Incline[rad] : Inport  Port=2
  Constant : Constant  Value=Vehicle.Mass
  Constant1 : Constant  Value=Vehicle.COG.Front
  Constant2 : Constant  Value=Vehicle.COG.Rear
  Constant3 : Constant  Value=Environment.g
  Constant4 : Constant  Value=Vehicle.COG.Height
  Divide : Product  Inputs=*/
  G*vzdalenost od predni napr. : Product
  Memory : Memory  X0=Vehicle.Mass/2
  Memory1 : Memory  X0=Vehicle.Mass/2
  Product : Product
  Product1 : Product
  Subtract : Sum  Inputs=+++
  Subtract1 : Sum  Inputs=+-
  Sum1 : Sum
  To Workspace2 : ToWorkspace  VariableName=Fn_Wheel_R  SampleTime=t_sample  SaveFormat=Array
  To Workspace3 : ToWorkspace  VariableName=Fn_Wheel_F  SampleTime=t_sample  SaveFormat=Array
  Trigonometric Function : Trigonometry  Operator=cos
  Trigonometric Function1 : Trigonometry
  m*a*vyska teziste : Product  Inputs=3
  m*g : Product
  m*g1 : Product
  Fn_Wheel_F : Outport
  Fn_Wheel_R : Outport  Port=2
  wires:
  acc/1 -> m*a*vyska teziste/1
  Product1/1 -> Subtract/3
  m*g1/1 -> Product1/1
  Product/1 -> Subtract/2
  Memory1/1 -> Fn_Wheel_R/1, To Workspace2/1
  Memory/1 -> Fn_Wheel_F/1, To Workspace3/1
  Constant/1 -> m*a*vyska teziste/2, m*g/1
  Constant3/1 -> m*g/2
  Constant1/1 -> G*vzdalenost od predni napr./2, Sum1/1
  Constant2/1 -> Sum1/2
  Sum1/1 -> Divide/2
  Constant4/1 -> m*g1/1, m*a*vyska teziste/3
  m*a*vyska teziste/1 -> Subtract/1
  G*vzdalenost od predni napr./1 -> Product/1
  m*g/1 -> m*g1/2, Subtract1/1, G*vzdalenost od predni napr./1
  Subtract/1 -> Divide/1
  Divide/1 -> Memory1/1, Subtract1/2
  Subtract1/1 -> Memory/1
  Road_Incline[rad]/1 -> Trigonometric Function/1, Trigonometric Function1/1
  Trigonometric Function/1 -> Product/2
  Trigonometric Function1/1 -> Product1/2

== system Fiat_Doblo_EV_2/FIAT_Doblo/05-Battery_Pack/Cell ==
  Current [A] : Inport
  Charging : Subsystem
  Compare To Constant : simulink/Logic and Bit Operations/Compare To Constant  relop=>=  const=0  OutDataTypeStr=uint8
  Demux : Demux  Outputs=2
  Discharging : Subsystem
  Mux : Mux  Inputs=2
  Mux1 : Mux  Inputs=2
  SOC calculations Ah : Subsystem
  Switch : Switch
  Thermo-model : Subsystem
  U_terminal [V] : Outport
  P_loss [w] : Outport  Port=2
  SOC[%] : Outport  Port=3
  T_cell[C] : Outport  Port=4
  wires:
  Demux/2 -> Thermo-model/1(P_loss [W]), P_loss [w]/1
  Demux/1 -> U_terminal [V]/1
  Switch/1 -> Demux/1
  Discharging/2(P_loss[W]) -> Mux1/2
  Discharging/1(U_terminal [V]) -> Mux1/1
  Mux1/1 -> Switch/3
  Mux/1 -> Switch/1
  Compare To Constant/1 -> Switch/2
  Charging/2(P_loss[W]) -> Mux/2
  Charging/1(U_terminal [V]) -> Mux/1
  Thermo-model/1(T_cell[C]) -> T_cell[C]/1, Discharging/1(Temperature), Charging/1(Temperature)
  SOC calculations Ah/1(SOC) -> SOC[%]/1, Charging/2(SOC), Discharging/2(SOC)
  Current [A]/1 -> Discharging/3(Current_Cell [A]), Charging/3(Current_Cell [A]), SOC calculations Ah/1(Current [A]), Compare To Constant/1

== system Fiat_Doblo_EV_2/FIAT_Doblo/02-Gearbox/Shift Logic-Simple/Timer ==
  Set : Inport
  Reset : Inport  Port=2
  Add1 : Sum  Inputs=-+
  Clock : Clock
  Memory : Memory
  S-R Flip-Flop : simulink_extras/Flip Flops/S-R Flip-Flop  initial_condition=0
  Switch1 : Switch  Threshold=1
  Terminator_1 : Terminator
  Count : Outport
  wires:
  S-R Flip-Flop/2 -> Terminator_1/1
  Reset/1 -> S-R Flip-Flop/2
  S-R Flip-Flop/1 -> Switch1/2
  Set/1 -> S-R Flip-Flop/1
  Add1/1 -> Count/1
  Clock/1 -> Switch1/3, Add1/2
  Memory/1 -> Switch1/1, Add1/1
  Switch1/1 -> Memory/1

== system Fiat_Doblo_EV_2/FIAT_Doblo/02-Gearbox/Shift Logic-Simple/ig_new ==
  ig : Inport
  Trigger : TriggerPort
  Data Store Write1 : DataStoreWrite  DataStoreName=ig_new
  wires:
  ig/1 -> Data Store Write1/1

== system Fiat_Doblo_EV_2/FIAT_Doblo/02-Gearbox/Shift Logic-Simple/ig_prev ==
  ig : Inport
  Trigger : TriggerPort
  Data Store Write1 : DataStoreWrite  DataStoreName=ig_prev
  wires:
  ig/1 -> Data Store Write1/1

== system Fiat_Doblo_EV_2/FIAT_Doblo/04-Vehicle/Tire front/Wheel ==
  F_tire : Inport
  T_drsft : Inport  Port=2
  "        " : Gain  Gain=2*Vehicle.Tyre.Front.Rdyn
  " Inertia Wheel" : Gain  Gain=1/(2*Vehicle.Tyre.Rear.Inertia)
  Sum10 : Sum  Inputs=|-|+|
  "to Rot Speed     " : Integrator  InitialCondition=omric
  om_wheel : Outport
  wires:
  "to Rot Speed     "/1 -> om_wheel/1  "om_wheel [rad/s]"
  "        "/1 -> Sum10/1  "T_tire"
  T_drsft/1 -> Sum10/2  "T_drv_sft"
  F_tire/1 -> "        "/1
  " Inertia Wheel"/1 -> "to Rot Speed     "/1
  Sum10/1 -> " Inertia Wheel"/1

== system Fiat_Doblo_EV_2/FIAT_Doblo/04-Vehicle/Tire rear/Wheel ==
  F_tire : Inport
  T_drsft : Inport  Port=2
  "        " : Gain  Gain=2*Vehicle.Tyre.Front.Rdyn
  " Inertia Wheel" : Gain  Gain=1/(2*Vehicle.Tyre.Front.Inertia)
  Sum10 : Sum  Inputs=|-|+|
  "to Rot Speed     " : Integrator  InitialCondition=omric
  om_wheel : Outport
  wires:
  Sum10/1 -> " Inertia Wheel"/1
  " Inertia Wheel"/1 -> "to Rot Speed     "/1
  F_tire/1 -> "        "/1
  T_drsft/1 -> Sum10/2  "T_drv_sft"
  "        "/1 -> Sum10/1  "T_tire"
  "to Rot Speed     "/1 -> om_wheel/1  "om_wheel [rad/s]"

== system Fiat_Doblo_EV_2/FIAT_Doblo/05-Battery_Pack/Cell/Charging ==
  Temperature : Inport
  SOC : Inport  Port=2
  Current_Cell [A] : Inport  Port=3
  Add : Sum  Inputs=+-
  IR-Chrg : Lookup_n-D  BreakpointsForDimension1=BatteryData.Chrg.IR.Vektor_Temp  BreakpointsForDimension2=BatteryData.Chrg.IR.Vektor_SOC  Table=BatteryData.Chrg.IR.Data/1000  RndMeth=Simplest
  OCV-Chrg : Lookup_n-D  BreakpointsForDimension1=BatteryData.Chrg.OCV.Vektor_Temp  BreakpointsForDimension2=BatteryData.Chrg.OCV.Vektor_SOC  Table=BatteryData.Chrg.OCV.Data  RndMeth=Simplest
  Product : Product
  Product1 : Product
  U_terminal [V] : Outport
  P_loss[W] : Outport  Port=2
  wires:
  Product1/1 -> P_loss[W]/1
  Add/1 -> U_terminal [V]/1
  Product/1 -> Product1/1, Add/2
  Current_Cell [A]/1 -> Product1/2, Product/2
  IR-Chrg/1 -> Product/1
  OCV-Chrg/1 -> Add/1
  SOC/1 -> IR-Chrg/2, OCV-Chrg/2
  Temperature/1 -> IR-Chrg/1, OCV-Chrg/1

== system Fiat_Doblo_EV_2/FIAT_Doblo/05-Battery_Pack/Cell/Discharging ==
  Temperature : Inport
  SOC : Inport  Port=2
  Current_Cell [A] : Inport  Port=3
  Add : Sum  Inputs=+-
  IR-Dchrg : Lookup_n-D  BreakpointsForDimension1=BatteryData.Dchrg.IR.Vektor_Temp  BreakpointsForDimension2=BatteryData.Dchrg.IR.Vektor_SOC  Table=BatteryData.Dchrg.IR.Data/1000  RndMeth=Simplest
  OCV-Dchrg : Lookup_n-D  BreakpointsForDimension1=BatteryData.Chrg.OCV.Vektor_Temp  BreakpointsForDimension2=BatteryData.Chrg.OCV.Vektor_SOC  Table=BatteryData.Chrg.OCV.Data  RndMeth=Simplest
  Product1 : Product
  Product2 : Product
  U_terminal [V] : Outport
  P_loss[W] : Outport  Port=2
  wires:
  OCV-Dchrg/1 -> Add/1
  Product2/1 -> P_loss[W]/1
  Add/1 -> U_terminal [V]/1
  Product1/1 -> Product2/1, Add/2
  Current_Cell [A]/1 -> Product2/2, Product1/2
  IR-Dchrg/1 -> Product1/1
  SOC/1 -> OCV-Dchrg/2, IR-Dchrg/2
  Temperature/1 -> OCV-Dchrg/1, IR-Dchrg/1

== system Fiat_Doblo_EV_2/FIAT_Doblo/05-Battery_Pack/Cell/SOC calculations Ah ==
  Current [A] : Inport
  Add1 : Sum  Inputs=+-
  Add2 : Sum  Inputs=-+
  Add3 : Sum  Inputs=+-
  Capacity [Ah] : Constant  Value=Battery.Cell.Capacity
  Divide2 : Product  Inputs=*/
  Gain : Gain  Gain=1/100
  Gain1 : Gain  Gain=3600
  Gain2 : Gain  Gain=100
  Integrator1 : Integrator
  Konst : Constant  Value=100
  Product : Product
  SOCinit : Constant  Value=Battery.SOC.Init
  SOC : Outport
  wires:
  Add2/1 -> Divide2/1
  Divide2/1 -> Gain2/1
  Product/1 -> Divide2/2, Add2/2
  Integrator1/1 -> Add2/1
  SOCinit/1 -> Gain/1, Add3/2
  Gain1/1 -> Product/2
  Capacity [Ah]/1 -> Gain1/1
  Current [A]/1 -> Integrator1/1
  Gain2/1 -> Add1/1
  Add1/1 -> SOC/1
  Gain/1 -> Product/1
  Konst/1 -> Add3/1
  Add3/1 -> Add1/2

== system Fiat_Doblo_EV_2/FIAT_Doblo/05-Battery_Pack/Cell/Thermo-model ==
  P_loss [W] : Inport
  Temp : Constant  Value=Battery.Cell.Temp
  Terminator : Terminator
  T_cell[C] : Outport
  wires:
  P_loss [W]/1 -> Terminator/1
  Temp/1 -> T_cell[C]/1
